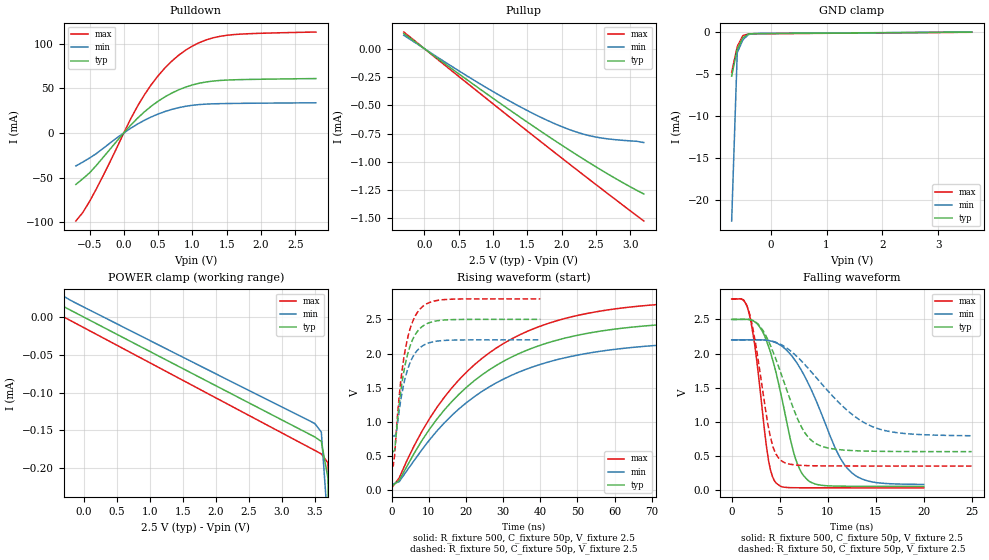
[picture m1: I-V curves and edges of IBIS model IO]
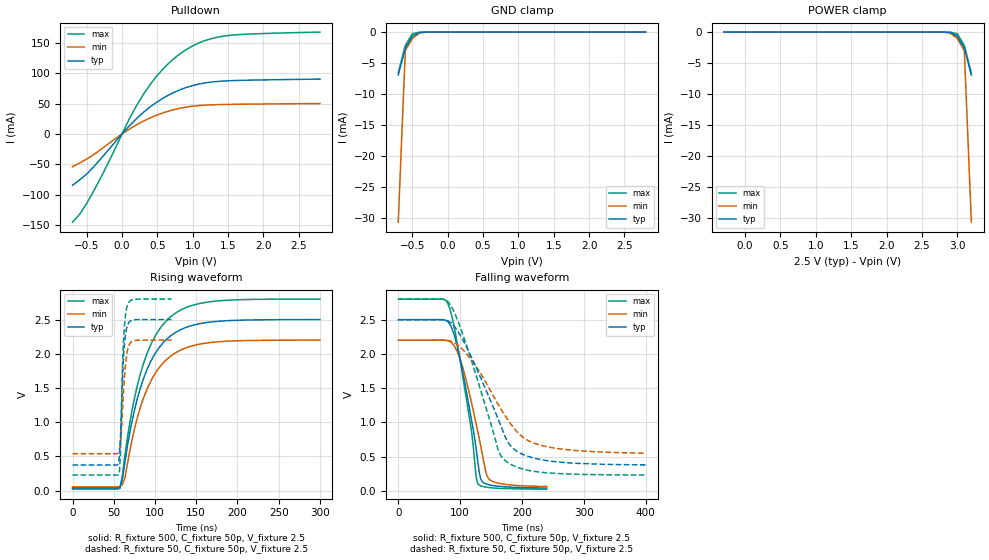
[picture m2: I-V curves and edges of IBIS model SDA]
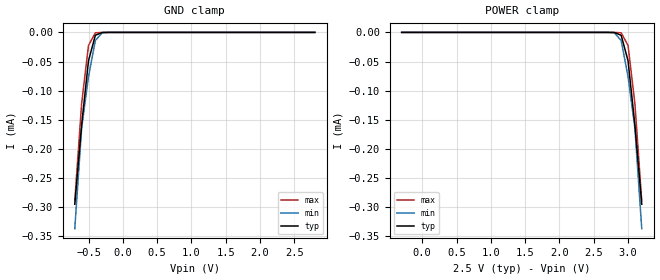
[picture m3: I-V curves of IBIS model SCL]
[IBIS Ver]   3.2
[Comment Char]   |_char
| VDD Nom: 2.5v, Min: 2.2v, Max: 2.8v
[File name]   pca9673_2_5v.ibs
[File Rev]   1
[Date]   08-25-2008
[Source]
[Notes]
[Disclaimer]
(C) Copyright 2007 NXP Semiconductors
All rights reserved
NXP Semiconductors (NXP) does not warrant that this model and any other
accompanying information (Model) accurately or fully represents the
operating characteristics and specifications of the semiconductor
products to which the Model relates.  Moreover, the Model is furnished
on an "as is" and with "all faults" basis, and without support or
warranty of any kind.  NXP disclaims all warranties, whether expressed
or implied or statutory, including without limitation all implied
warranties of non-infringement, merchantability and fitness for any
purpose, and those arising from a course of dealing or usage of trade.
NXP does not convey any license under its or any third party's patents,
copyrights or other intellectual property or proprietary rights.
You and your company assume any and all risks and liability arising out
of the application or use of the Model.
In no event shall NXP be liable for any direct, indirect, special,
consequential or incidental damages, however caused, whether in
warranty, contract or tort (including negligence), strict liability or
other legal theory, including, without limitation, for lost profits,
business interruption, or corruption or loss of data or information,
arising out of or in connection with the use of or the inability to use
the Model, even if NXP has been advised of the possibility of such
damages.
NXP provides the Model as a courtesy to our customers. You and your
company shall not distribute, convey, sell, or give the Model to anyone
else without receiving prior written permission from NXP.
NXP reserves the right to make changes without notice to the Model to
improve reliability, function, or design.
Please be aware that your receipt and subsequent use of the Model shall
serve as acceptance of these terms and conditions.  If you do not
accept these terms, return or destroy the Model immediately.
[Copyright]
2008
| SO24 package
[Component]   PCA9673D
Si_location Pin
Timing_location Pin
[Manufacturer]   NXP Semiconductors
[Package]
R_pkg   0.14   0.12   0.18
L_pkg   5.71n   3.95n   7.95n
C_pkg   1.01p   0.72p   1.49p
[Pin] signal_name   model_name   R_pin   L_pin   C_pin
1   INTb   INT   0.18   6.01n   0.97p
2   AD1   ADDR   0.14   7.94n   1.21p
3   RST   ADDR   0.16   7.06n   1.32p
4   P00   IO   0.18   6.01n   1.07p
5   P01   IO   0.14   4.98n   0.88p
6   P02   IO   0.13   4.30n   0.80p
7   P03   IO   0.12   3.95n   0.74p
8   P04   IO   0.12   3.95n   0.72p
9   P05   IO   0.13   4.30n   0.76p
10   P06   IO   0.14   4.98n   0.85p
11   P07   IO   0.18   6.01n   0.97p
12   VSS   GND   0.16   7.06n   1.20p
13   P10   IO   0.14   7.95n   1.45p
14   P11   IO   0.14   7.95n   1.49p
15   P12   IO   0.16   7.06n   1.32p
16   P13   IO   0.18   6.01n   1.07p
17   P14   IO   0.14   4.98n   0.88p
18   P15   IO   0.13   4.30n   0.80p
19   P16   IO   0.12   3.95n   0.74p
20   P17   IO   0.12   3.95n   0.72p
21   AD0   ADDR   0.13   4.30n   0.76p
22   SCL   SCL   0.14   4.98n   0.85p
23   SDA   SDA   0.18   6.01n   0.97p
24   VDD   POWER   0.16   7.06n   1.20p
| TSSOP24 package
[Component]   PCA9673PW
Si_location Pin
Timing_location Pin
[Manufacturer]   NXP Semiconductors
[Package]
R_pkg   52.70m   31.50m   67.00m
L_pkg   2.19n   1.32n   3.39n
C_pkg   0.48p   0.35p   0.93p
[Pin] signal_name   model_name   R_pin   L_pin   C_pin
1   INTB   INT   66.40m   2.36n   0.47p
2   AD1   ADDR   66.10m   3.39n   0.57p
3   RST   ADDR   67.00m   2.94n   0.59p
4   P00   IO   66.40m   2.36n   0.47p
5   P01   IO   47.10m   1.67n   0.40p
6   P02   IO   38.00m   1.44n   0.37p
7   P03   IO   31.50m   1.32n   0.35p
8   P04   IO   31.50m   1.32n   0.35p
9   P05   IO   38.00m   1.44n   0.37p
10   P06   IO   47.10m   1.67n   0.40p
11   P07   IO   66.40m   2.36n   0.47p
12   VSS   GND   67.00m   2.94n   0.59p
13   P10   IO   66.10m   3.39n   0.61p
14   P11   IO   66.20m   3.39n   0.61p
15   P12   IO   67.00m   2.94n   0.59p
16   P13   IO   66.50m   2.36n   0.47p
17   P14   IO   47.10m   1.67n   0.40p
18   P15   IO   38.00m   1.45n   0.37p
19   P16   IO   31.50m   1.32n   0.35p
20   P17   IO   31.50m   1.32n   0.35p
21   AD0   ADDR   38.00m   1.45n   0.37p
22   SCL   SCL   47.10m   1.67n   0.40p
23   SDA   SDA   66.50m   2.36n   0.47p
24   VDD   POWER   67.00m   2.94n   0.59p
| SSOP24
[Component]   PCA9673DB
Si_location Pin
Timing_location Pin
[Manufacturer]   NXP Semiconductors
[Package]
R_pkg   54.20m   39.70m   64.80m
L_pkg   2.55n   1.89n   3.58n
C_pkg   0.636p   0.52p   1.05p
[Pin] signal_name   model_name   R_pin   L_pin   C_pin
1   INTB   INT   63.00m   2.53n   0.58p
2   AD1   ADDR   61.20m   3.56n   0.70p
3   RST   ADDR   64.80m   3.10n   0.76p
4   P00   IO   63.00m   2.53n   0.60p
5   P01   IO   52.60m   2.17n   0.57p
6   P02   IO   43.90m   2.03n   0.56p
7   P03   IO   39.70m   1.89n   0.54p
8   P04   IO   39.70m   1.89n   0.52p
9   P05   IO   43.90m   2.03n   0.55p
10   P06   IO   52.60m   2.17n   0.56p
11   P07   IO   63.00m   2.53n   0.58p
12   VSS   GND   64.80m   3.10n   0.71p
13   P10   IO   61.20m   3.56n   1.01p
14   P11   IO   61.20m   3.56n   1.05p
15   P12   IO   64.80m   3.10n   0.80p
16   P13   IO   63.00m   2.53n   0.65p
17   P14   IO   52.60m   2.17n   0.59p
18   P15   IO   43.90m   2.03n   0.56p
19   P16   IO   39.70m   1.89n   0.54p
20   P17   IO   39.70m   1.89n   0.53p
21   AD0   ADDR   43.90m   2.03n   0.56p
22   SCL   SCL   52.60m   2.17n   0.57p
23   SDA   SDA   63.00m   2.53n   0.60p
24   VDD   POWER   64.80m   3.10n   0.76p
[Define Package Model]  HVQFN24
[Manufacturer]  ST-NXP Wireless
|[Simulated] Chris Hunat
|[Approved] Wayne Nunn, Roger Real
[OEM]  Unknown
[Description]  Full package model
[Number Of Pins]  23
[Pin Numbers]
pin1   | pin1 = lead1
pin2   | pin2 = lead2
pin3   | pin3 = lead3
pin4   | pin4 = lead4
pin5   | pin5 = lead5
pin6   | pin6 = lead6
pin7   | pin7 = lead7
pin8   | pin8 = lead8
pin9   | pin9 = lead9
pin10   | pin10 = lead10
pin11   | pin11 = lead11
pin12   | pin12 = lead12
pin13   | pin13 = lead13
pin14   | pin14 = lead14
pin15   | pin15 = lead15
pin17   | pin17 = lead17
pin18   | pin18 = lead18
pin19   | pin19 = lead19
pin20   | pin20 = lead20
pin21   | pin21 = lead21
pin22   | pin22 = lead22
pin23   | pin23 = lead23
pin24   | pin24 = lead24
[Model Data]
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[End Model Data]
[End Package Model]
[Define Package Model]  DHVQFN24
[Manufacturer]  ST-NXP Wireless
|[Simulated] Chris Hunat
|[Approved] Wayne Nunn, Roger Real
[OEM]  Unknown
[Description]  Full package model
[Number Of Pins]  24
[Pin Numbers]
|Pin Num   Terminal Name
1   | lead1:pin1
2   | lead2:pin2
3   | lead3:pin3
4   | lead4:pin4
5   | lead5:pin5
6   | lead6:pin6
7   | lead7:pin7
8   | lead8:pin8
9   | lead9:pin9
10   | lead10:pin10
11   | lead11:pin11
12   | lead12:pin12
13   | lead13:pin13
14   | lead14:pin14
15   | lead15:pin15
16   | lead16:pin16
17   | lead17:pin17
18   | lead18:pin18
19   | lead19:pin19
20   | lead20:pin20
21   | lead21:pin21
22   | lead22:pin22
23   | lead23:pin23
24   | lead24:pin24
[Model Data]
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[End Model Data]
[End Package Model]
| Models and submodels in the file (5): IO (I/O), SDA (I/O_open_drain), SCL (Input), ADDR (Input), INT (Open_drain)
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[Model]   IO
Model_type I/O
Vinh=1.5
Vinl=0.75
Vref=2.5
Vmeas=1.25
Rref=500
Cref=50p
C_comp   7p   6.8p   7.2p
[Model Spec]
Vinh   1.494   1.195   1.893
Vinl   1.023   0.854   1.563
[Temperature Range] 27   85   -40
[Voltage Range]   2.5   2.2   2.8
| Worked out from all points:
|   slope of the pulldown table from 0 to 0.375 V, typ, clamps not added: 13.3 ohm
|   slope of the pullup table from 0 to 0.375 V, typ, clamps not added: 2.25 kohm
|   GND clamp passes 1 mA (typ) near -0.52 V on its own axis
|   falling waveform, R_fixture 500, C_fixture 50p, V_fixture 2.5: 20-80 % time 2.41ns typ, 4ns min, 1.41ns max; typ from 2.5 V to 0.056 V
|   falling waveform, R_fixture 50, C_fixture 50p, V_fixture 2.5: 20-80 % time 3.12ns typ, 5.76ns min, 1.66ns max; typ from 2.5 V to 0.564 V
|   rising waveform, R_fixture 500, C_fixture 50p, V_fixture 2.5: 20-80 % time 28.7ns typ, 29.5ns min, 28ns max; typ from 0.055 V to 2.5 V
|   rising waveform, R_fixture 50, C_fixture 50p, V_fixture 2.5: 20-80 % time 3.52ns typ, 3.59ns min, 3.48ns max; typ from 0.564 V to 2.5 V
[Pullup]
-300mV    132.9uA    118uA      146.5uA
500mV     -221.6uA   -195uA     -244.5uA
1V        -438.3uA   -378.9uA   -487.1uA
1.5V      -648.9uA   -546.8uA   -727.5uA
1.9V      -811.8uA   -663.1uA   -918uA
2.2V      -929.9uA   -733.5uA   -1.06mA
2.5V      -1.044mA   -781.3uA   -1.2mA
2.9V      -1.186mA   -810.6uA   -1.386mA
3.2V      -1.284mA   -830uA     -1.523mA
[Pulldown]
-700mV    -57.71mA   -36.98mA   -98.68mA
-600mV    -51.44mA   -32.7mA    -89.33mA
-500mV    -44.74mA   -28.1mA    -76.78mA
-200mV    -18.1mA    -11.23mA   -32.15mA
100mV     8.746mA    5.272mA    15.89mA
300mV     23.67mA    14.2mA     42.8mA
500mV     35.58mA    21.22mA    64.11mA
800mV     48.34mA    28.35mA    87.14mA
1.1V      55.72mA    31.81mA    101.2mA
1.4V      58.81mA    32.83mA    108.3mA
1.8V      59.91mA    33.24mA    111.1mA
2.8V      60.93mA    33.79mA    113.1mA
[GND Clamp]
-700mV    -5.214mA   -22.45mA   -4.761mA
-600mV    -2.033mA   -2.422mA   -1.708mA
-500mV    -655.6uA   -909.6uA   -400.5uA
-400mV    -212.8uA   -276uA     -193uA
-200mV    -158.7uA   -141uA     -176.5uA
3.6V      13.62uA    27.33uA    109.1pA
[POWER Clamp]
-300mV    13.62uA    27.33uA    109.1pA
-100mV    4.551uA    17.65uA    -9.31uA
3.5V      -158.7uA   -141uA     -176.5uA
3.6V      -164.6uA   -152.1uA   -181.2uA
3.7V      -212.8uA   -276uA     -193uA
3.8V      -655.6uA   -909.6uA   -400.5uA
4V        -5.214mA   -22.45mA   -4.761mA
[Falling Waveform]
R_fixture=500
C_fixture=50p
V_fixture=2.5
V_fixture_min=2.2
V_fixture_max=2.8
0s        2.5V       2.2V       2.8V
1.818ns   2.499V     2.201V     2.589V
2.424ns   2.463V     2.201V     2.107V
3.838ns   2.104V     2.191V     436.2mV
4.646ns   1.707V     2.157V     102.3mV
6.465ns   546.4mV    1.928V     35.83mV
8.081ns   128.8mV    1.533V     34.45mV
10.91ns   59.6mV     580.2mV    34.05mV
12.53ns   57.13mV    252.8mV    34.02mV
20ns      55.55mV    84.44mV    34.01mV
[Falling Waveform]
R_fixture=50
C_fixture=50p
V_fixture=2.5
V_fixture_min=2.2
V_fixture_max=2.8
0s        2.5V       2.2V       2.8V
1.263ns   2.501V     2.2V       2.779V
1.768ns   2.5V       2.201V     2.632V
2.525ns   2.457V     2.201V     2.119V
4.04ns    2.119V     2.186V     774.4mV
5.051ns   1.745V     2.138V     442.8mV
7.323ns   911.6mV    1.883V     362.7mV
9.091ns   659.2mV    1.602V     355.9mV
14.9ns    569.9mV    917.3mV    353.7mV
25ns      564.3mV    797.1mV    353.7mV
[Rising Waveform]
R_fixture=500
C_fixture=50p
V_fixture=2.5
V_fixture_min=2.2
V_fixture_max=2.8
0s        55.5mV     81.08mV    34.01mV
2.02ns    145.4mV    125.5mV    180.6mV
6.061ns   541.7mV    435.7mV    652.6mV
10.1ns    887.5mV    731.6mV    1.041V
20.2ns    1.51V      1.285V     1.732V
32.32ns   1.95V      1.683V     2.215V
46.46ns   2.223V     1.936V     2.51V
62.63ns   2.374V     2.077V     2.67V
86.87ns   2.461V     2.161V     2.761V
200ns     2.5V       2.2V       2.8V
[Rising Waveform]
R_fixture=50
C_fixture=50p
V_fixture=2.5
V_fixture_min=2.2
V_fixture_max=2.8
0s        564.2mV    792.2mV    353.7mV
404ps     564.2mV    792.2mV    353.7mV
808.1ps   586.5mV    792.4mV    526.5mV
1.212ns   815.1mV    836.7mV    855.6mV
2.02ns    1.266V     1.169V     1.385V
3.636ns   1.843V     1.646V     2.057V
5.253ns   2.157V     1.904V     2.414V
7.677ns   2.37V      2.087V     2.655V
14.14ns   2.49V      2.191V     2.789V
40ns      2.5V       2.2V       2.8V
[Ramp]
R_load=500
dV/dt_r   2.854E-1/1.585E-9   2.173E-1/3.221E-9   3.507E-1/9.177E-10
dV/dt_f   1.467E+0/7.289E-10   1.271E+0/1.459E-9   1.660E+0/3.514E-10
|[End   IO
| [End   SDA
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[Model]   SDA
Model_type I/O_open_drain
Vinh=1.5
Vinl=0.75
Vref=2.5
Vmeas=1.25
Rref=1k
Cref=50p
C_comp   6p   5.8p   6.2p
[Model Spec]
[Temperature Range] 27   85   -40
[Voltage Range]   2.5   2.2   2.8
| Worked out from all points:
|   slope of the pulldown table from 0 to 0.375 V, typ, clamps not added: 8.82 ohm
|   GND clamp passes 1 mA (typ) near -0.52 V on its own axis
|   falling waveform, R_fixture 500, C_fixture 50p, V_fixture 2.5: 20-80 % time 29.1ns typ, 31.6ns min, 28.4ns max; typ from 2.5 V to 0.041 V
|   falling waveform, R_fixture 50, C_fixture 50p, V_fixture 2.5: 20-80 % time 60.6ns typ, 68.7ns min, 52.9ns max; typ from 2.5 V to 0.379 V
|   rising waveform, R_fixture 500, C_fixture 50p, V_fixture 2.5: 20-80 % time 35.4ns typ, 35.5ns min, 35.3ns max; typ from 0.037 V to 2.5 V
|   rising waveform, R_fixture 50, C_fixture 50p, V_fixture 2.5: 20-80 % time 4.34ns typ, 5.3ns min, 3.79ns max; typ from 0.374 V to 2.5 V
[Pulldown]
-700mV    -84.71mA   -54.07mA   -145.5mA
-600mV    -75.81mA   -47.97mA   -132.5mA
-400mV    -54.01mA   -34.18mA   -93.93mA
-200mV    -27.3mA    -16.82mA   -48.96mA
100mV     13.05mA    7.75mA     24.12mA
300mV     35.44mA    21.05mA    64.86mA
500mV     53.16mA    31.45mA    96.69mA
800mV     71.93mA    41.95mA    130.5mA
1.1V      82.63mA    47.01mA    150.8mA
1.4V      87.08mA    48.54mA    160.7mA
1.8V      88.74mA    49.21mA    164.8mA
2.8V      90.48mA    50.19mA    168mA
[GND Clamp]
-700mV    -6.935mA   -30.66mA   -6.593mA
-600mV    -2.591mA   -2.99mA    -2.148mA
-500mV    -653.7uA   -1.019mA   -278.6uA
-400mV    -54.45uA   -160.3uA   -7.607uA
-300mV    -1.471uA   -7.716uA   -80.08nA
2.8V      157.3pA    305.4pA    145.7pA
[POWER Clamp]
-300mV    157.3pA    305.4pA    145.7pA
2.8V      -1.471uA   -7.716uA   -80.08nA
2.9V      -54.45uA   -160.3uA   -7.607uA
3V        -653.7uA   -1.019mA   -278.6uA
3.1V      -2.591mA   -2.99mA    -2.148mA
3.2V      -6.935mA   -30.66mA   -6.593mA
[Falling Waveform]
R_fixture=500
C_fixture=50p
V_fixture=2.5
V_fixture_min=2.2
V_fixture_max=2.8
0s        2.5V       2.2V       2.8V
80ns      2.472V     2.193V     2.74V
99.39ns   1.951V     1.941V     1.942V
118.8ns   1.019V     1.274V     848.5mV
126.1ns   607.3mV    972.7mV    196.4mV
128.5ns   436.1mV    869.8mV    106.9mV
133.3ns   173.8mV    656.4mV    73.17mV
140.6ns   105.3mV    313.9mV    55.45mV
147.9ns   85.93mV    161mV      46.3mV
240ns     41.13mV    62.75mV    24.28mV
[Falling Waveform]
R_fixture=50
C_fixture=50p
V_fixture=2.5
V_fixture_min=2.2
V_fixture_max=2.8
0s        2.5V       2.2V       2.8V
72.73ns   2.499V     2.2V       2.799V
84.85ns   2.458V     2.187V     2.709V
96.97ns   2.323V     2.126V     2.469V
117.2ns   1.975V     1.924V     1.937V
161.6ns   1.047V     1.262V     590.7mV
177.8ns   705mV      1.029V     409.4mV
202ns     529.7mV    778.9mV    316.6mV
234.3ns   450mV      657mV      268.4mV
400ns     378.9mV    550.1mV    230.6mV
[Rising Waveform]
R_fixture=500
C_fixture=50p
V_fixture=2.5
V_fixture_min=2.2
V_fixture_max=2.8
0s        36.68mV    54.25mV    22.15mV
57.58ns   54.78mV    61.72mV    33.04mV
60.61ns   170.3mV    93.88mV    241.5mV
63.64ns   427.5mV    189.4mV    527.6mV
72.73ns   1.047V     777.1mV    1.209V
84.85ns   1.596V     1.313V     1.811V
100ns     2.001V     1.709V     2.255V
121.2ns   2.283V     1.986V     2.563V
169.7ns   2.468V     2.168V     2.765V
300ns     2.5V       2.2V       2.8V
[Rising Waveform]
R_fixture=50
C_fixture=50p
V_fixture=2.5
V_fixture_min=2.2
V_fixture_max=2.8
0s        374mV      540mV      228.7mV
55.76ns   413.9mV    557.3mV    231.5mV
56.97ns   521mV      604mV      294mV
58.18ns   798.5mV    699.6mV    550.7mV
60.61ns   1.636V     1.168V     1.825V
61.82ns   1.954V     1.448V     2.191V
64.24ns   2.289V     1.833V     2.566V
66.67ns   2.419V     2.052V     2.71V
73.94ns   2.495V     2.191V     2.795V
120ns     2.5V       2.2V       2.8V
[Ramp]
R_load=500
dV/dt_r   1.478E+0/1.583E-9   1.463E+0/2.880E-9   1.488E+0/9.563E-10
dV/dt_f   1.476E+0/2.825E-8   1.457E+0/3.507E-8   1.487E+0/2.413E-8
|[End   SDA
| [End   SCL
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[Model]   SCL
Model_type Input
Vinh=1.5
Vinl=0.75
C_comp   5p   4.8p   5.2p
[Model Spec]
Vinh   2.31   1.61   3.85
Vinl   0.99   0.69   1.65
[Temperature Range] 27   85   -40
[Voltage Range]   2.5   2.2   2.8
[GND Clamp]
-700mV    -295uA     -337uA     -289.5uA
-600mV    -158.8uA   -164.3uA   -122uA
-500mV    -48.62uA   -75.94uA   -22.35uA
-400mV    -4.926uA   -13.83uA   -710.6nA
-300mV    -138.4nA   -722.3nA   -7.551nA
2.8V      6.71pA     20.63pA    5.609pA
[POWER Clamp]
-300mV    6.71pA     20.63pA    5.609pA
2.8V      -138.4nA   -722.3nA   -7.551nA
2.9V      -4.926uA   -13.83uA   -710.6nA
3V        -48.62uA   -75.94uA   -22.35uA
3.1V      -158.8uA   -164.3uA   -122uA
3.2V      -295uA     -337uA     -289.5uA
